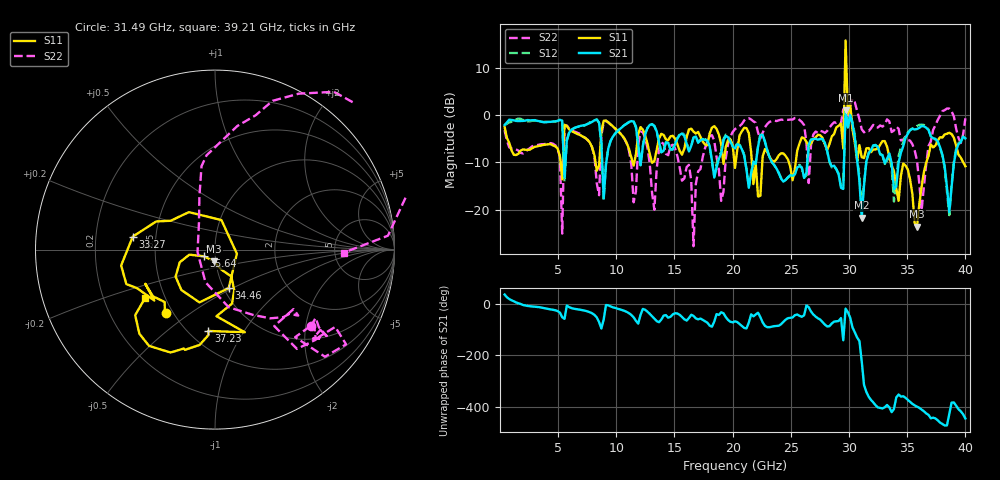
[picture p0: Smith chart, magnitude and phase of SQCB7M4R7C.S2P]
! Network Analyzer HP8722ES.07.66: Jul 25, 2000 Serial No. US39175408
! 26 Oct 2004  14:58:29
! Frequency  S11  S21  S12  S22
# HZ  S  DB R  50
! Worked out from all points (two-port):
!   201 points, 400 MHz to 40 GHz, reference 50 ohm
!   highest |S21| = 1.04 dB at 29.7 GHz (marker M1); lowest = -21.7 dB at 31.09 GHz (marker M2)
!   |S21| within 3 dB of the highest: 449.5 MHz to 5.363 GHz (4.913 GHz wide, 169 % of centre); 7.456 GHz to 8.534 GHz (1.079 GHz wide, 13.5 % of centre)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
!   lowest |S11| = -23.6 dB at 35.84 GHz (marker M3), VSWR 1.14, Z = 49.1 - j6.52 ohm
!   |S11| at or under -10 dB: 21.65 GHz to 22.55 GHz (896.7 MHz wide, 4.06 % of centre); 24.83 GHz to 25.42 GHz (589 MHz wide, 2.34 % of centre); 33.6 GHz to 36.64 GHz (3.039 GHz wide, 8.66 % of centre)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
!   |S22| runs from -27.7 to 3.5 dB; largest |S21 - S12| = 0.57
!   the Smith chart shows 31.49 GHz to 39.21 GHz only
!   S11 on the Smith chart (normalised r, x): 31.49 GHz: 0.46, -0.41; 33.27 GHz: 0.37, +0.07; 34.46 GHz: 1.05, -0.48; 35.64 GHz: 0.88, -0.07; 37.23 GHz: 0.62, -0.71; 39.21 GHz: 0.39, -0.27
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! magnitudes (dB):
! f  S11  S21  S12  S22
! 400 MHz  -2.5  -2.1  -2.2  -3.2
! 4.954 GHz  -7.1  -1.2  -1.2  -7.1
! 5.35 GHz  -13.6  -1.2  -1.2  -25.1
! 5.548 GHz  -2.1  -13.2  -14.1  -2.5
! 7.132 GHz  -4.6  -2.2  -2.3  -4.5
! 13.67 GHz  -5.0  -5.7  -5.8  -7.3
! 16.64 GHz  -3.5  -4.8  -4.7  -27.7
! 20.2 GHz  -11.2  -7.1  -6.7  -3.0
! 26.93 GHz  -5.2  -5.1  -5.0  -4.1
! 29.51 GHz  -7.1  -15.6  -14.2  1.2
! 29.7 GHz  15.8  1.0  0.6  -2.1
! 31.09 GHz  -8.9  -21.7  -19.0  -3.0
! 31.49 GHz  -7.0  -9.8  -9.8  -3.3
! 33.27 GHz  -6.7  -9.2  -9.6  -0.9
! 33.47 GHz  -8.8  -8.1  -8.7  -1.4
! 34.46 GHz  -12.9  -8.0  -6.9  -5.4
! 35.64 GHz  -22.9  -3.0  -2.7  -7.5
! 35.84 GHz  -23.6  -2.9  -2.3  -9.6
! 37.23 GHz  -6.8  -4.9  -4.8  -3.1
! 38.61 GHz  -3.7  -20.5  -21.2  1.4
! 39.21 GHz  -6.5  -7.4  -7.1  -2.9
! 40 GHz  -10.8  -4.9  -5.0  -0.7
